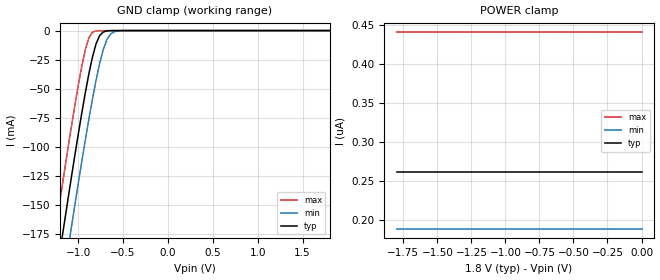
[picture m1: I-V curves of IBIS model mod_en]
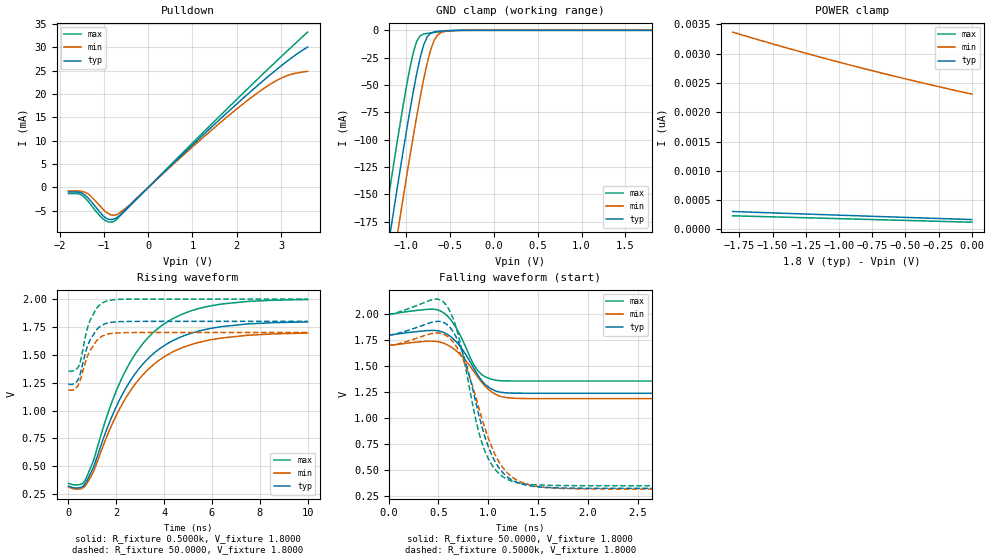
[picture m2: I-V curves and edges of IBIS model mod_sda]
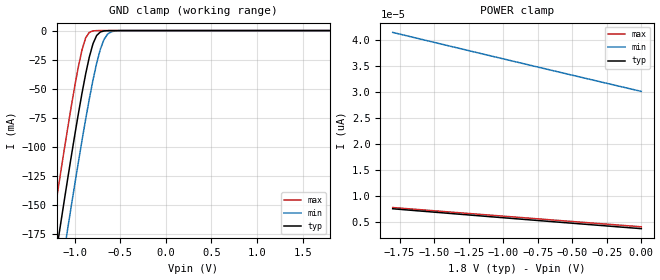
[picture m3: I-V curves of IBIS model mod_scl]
| IBIS (I/O, Buffer, Information, Specification) Model, officially
| electronic behavioral standard for Buffer structures of digital pins.
[IBIS ver]  4.0
[File name] m24c32_fd1_tssop8.ibs
[File Rev]  1.0
[Date]   2 March 2015
[Source]   CAD & Design Services (Catania) - STMicroelectronics
[Notes]
   (Note1)  This IBIS model includes the TSSOP8 package data
   (Note2)  This IBIS model has some Notes about the non-monotonicity
   of the I-V curves, but they are not indicative of problems
   inside the model;
[Copyright] (c) 2015 STMicroelectronics
|   Component M24C32
[Component] M24C32
[Manufacturer] STMicroelectronics
[Package]
| variable   typ   min   max
R_pkg   0.0   0.0   0.0
L_pkg   0.0H   0.0H   0.0H
C_pkg   0.0F   0.0F   0.0F
[Pin]   signal_name   model_name   R_pin   L_pin   C_pin
1   E1   mod_en   NA   NA   NA
2   E2   mod_en   NA   NA   NA
3   E3   mod_en   NA   NA   NA
4   VSS   GND   NA   NA   NA
5   SDA   mod_sda   NA   NA   NA
6   SCL   mod_scl   NA   NA   NA
7   WC   mod_wc   NA   NA   NA
8   VCC   POWER   NA   NA   NA
[Package Model]  182696_TSSOP8
[Define Package Model]  182696_TSSOP8
[Manufacturer]  STMicroelectronics
[OEM]  STMicroelectronics
[Description]  8 pin TSSOP package
[Number Of Pins]  8
[Pin Numbers]
|Pin Num   Terminal Name
1   | net1
2   | net2
3   | net3
4   | net4_GND
5   | net5
6   | net6
7   | net7
8   | net8_VDD
[Model Data]
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[End Model Data]
[End Package Model]
| Models and submodels in the file (4): mod_en (Input), mod_sda (I/O_open_drain), mod_scl (Input), mod_wc (Input)
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|   Model mod_en
[Model]   mod_en
Model_type Input
Vinl   =   0.540V
Vinh   =   1.260V
C_comp   1.763pF   1.683pF   1.933pF
[Temperature Range]  25.0000   85.0000   -40.0000
[Voltage Range]   1.8000V   1.7000V   2.0000V
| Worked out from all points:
|   GND clamp passes 1 mA (typ) near -0.71 V on its own axis
[GND_clamp]
|Voltage   I(typ)   I(min)   I(max)
-1.8V     -506.7mA   -549.3mA   -463.8mA
-1.28V    -230.6mA   -274mA     -186.5mA
-1.24V    -209.8mA   -253.3mA   -165.8mA
-1.16V    -168.9mA   -212.2mA   -124.8mA
-1.08V    -128.7mA   -171.8mA   -85.14mA
-920mV    -53.64mA   -94.29mA   -16.44mA
-840mV    -22.68mA   -58.76mA   -1.468mA
-800mV    -11.31mA   -42.6mA    -261.9uA
-720mV    -1.249mA   -16.25mA   -6.98uA
-680mV    -318.6uA   -7.797mA   -1.128uA
-600mV    -18.77uA   -1.043mA   -29.45nA
1.8V      3.674pA    30.76pA    3.627pA
[POWER_clamp]
|Voltage   I(typ)   I(min)   I(max)
-1.8V     261.2nA    189.1nA    440.6nA
-1.78V    261.2nA    189.1nA    440.6nA
-1.76V    261.2nA    189.1nA    440.6nA
0V        261.2nA    189.1nA    440.6nA
|   Model mod_sda
[Model]   mod_sda
Model_type I/O_open_drain
Polarity   Inverting
Vinl   =   0.540V
Vinh   =   1.260V
Vmeas  =   0.900V
Cref   =   10pF
Rref   =   1k
Vref   =   1.800V
C_comp   1.845pF   1.762pF   2.023pF
[Temperature Range]  25.0000   85.0000   -40.0000
[Voltage Range]   1.8000V   1.7000V   2.0000V
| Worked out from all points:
|   slope of the pulldown table from 0 to 0.27 V, typ, clamps not added: 109 ohm
|   GND clamp passes 1 mA (typ) near -0.65 V on its own axis
|   rising waveform, R_fixture 0.5000k, V_fixture 1.8000: 20-80 % time 2.25ns typ, 2.31ns min, 2.17ns max; typ from 0.322 V to 1.79 V
|   rising waveform, R_fixture 50.0000, V_fixture 1.8000: 20-80 % time 545ps typ, 565ps min, 512ps max; typ from 1.24 V to 1.8 V
|   falling waveform, R_fixture 50.0000, V_fixture 1.8000: 20-80 % time 225ps typ, 254ps min, 198ps max; typ from 1.8 V to 1.24 V
|   falling waveform, R_fixture 0.5000k, V_fixture 1.8000: 20-80 % time 266ps typ, 296ps min, 236ps max; typ from 1.8 V to 0.322 V
[Pulldown]
|Voltage   I(typ)   I(min)   I(max)
-1.8V     -956.6uA   -736.7uA   -1.299mA
-1.56V    -1.02mA    -766uA     -1.377mA
-1.38V    -2.037mA   -1.217mA   -2.706mA
-1.02V    -6.05mA    -4.667mA   -6.729mA
-900mV    -6.803mA   -5.579mA   -7.367mA
-780mV    -6.779mA   -5.962mA   -7.317mA
-660mV    -6.106mA   -5.539mA   -6.328mA
-480mV    -4.437mA   -4.234mA   -4.601mA
1.2V      10.89mA    10.37mA    11.4mA
2.4V      21.26mA    19.77mA    22.56mA
3.06V     26.48mA    23.66mA    28.53mA
3.6V      30.07mA    24.87mA    33.28mA
[GND_clamp]
|Voltage   I(typ)   I(min)   I(max)
-1.8V     -518.5mA   -561.2mA   -477.1mA
-1.28V    -237.2mA   -280.6mA   -194.5mA
-1.24V    -216mA     -259.5mA   -173.3mA
-1.16V    -174.3mA   -217.7mA   -131.6mA
-1.08V    -133.3mA   -176.5mA   -91.09mA
-920mV    -56.72mA   -97.5mA    -20.77mA
-840mV    -25.03mA   -61.28mA   -5.008mA
-800mV    -13.32mA   -44.79mA   -3.408mA
-720mV    -2.603mA   -17.83mA   -2.376mA
-680mV    -1.384mA   -9.107mA   -1.989mA
-600mV    -612.9uA   -1.891mA   -1.25mA
1.8V      166.6pA    2.361nA    109.5pA
[POWER_clamp]
|Voltage   I(typ)   I(min)   I(max)
-1.8V     304.6pA    3.37nA     231.1pA
-1.36V    269.7pA    3.079nA    204.3pA
-920mV    235.6pA    2.809nA    177.5pA
-480mV    202.2pA    2.561nA    150.8pA
0V        166.6pA    2.311nA    121.7pA
[Ramp]
| variable   typ   min   max
dV/dt_r   0.3370/0.5861n   0.3078/0.6032n   0.3862/0.5628n
dV/dt_f   0.3368/0.2838n   0.3075/0.2962n   0.3859/0.2619n
R_load = 50.0000
[Rising Waveform]
R_fixture= 0.5000k
V_fixture= 1.8000
V_fixture_min= 1.7000
V_fixture_max= 2.0000
|time   V(typ)   V(min)   V(max)
0s        321.8mV    314.6mV    346.1mV
700ps     344.7mV    324.2mV    376.4mV
1.05ns    494.1mV    454.1mV    554.7mV
1.75ns    912.3mV    841.1mV    1.038V
2.25ns    1.143V     1.059V     1.298V
2.95ns    1.376V     1.281V     1.555V
3.79ns    1.551V     1.451V     1.744V
4.79ns    1.668V     1.566V     1.867V
5.95ns    1.737V     1.635V     1.939V
10ns      1.795V     1.695V     1.996V
[Rising Waveform]
R_fixture= 50.0000
V_fixture= 1.8000
V_fixture_min= 1.7000
V_fixture_max= 2.0000
|time   V(typ)   V(min)   V(max)
0s        1.238V     1.187V     1.356V
220ps     1.24V      1.188V     1.359V
420ps     1.286V     1.234V     1.395V
520ps     1.352V     1.292V     1.461V
760ps     1.555V     1.467V     1.712V
920ps     1.638V     1.544V     1.815V
1.24ns    1.739V     1.64V      1.933V
1.62ns    1.784V     1.684V     1.983V
2.52ns    1.799V     1.699V     1.999V
10ns      1.8V       1.7V       2V
[Falling Waveform]
R_fixture= 50.0000
V_fixture= 1.8000
V_fixture_min= 1.7000
V_fixture_max= 2.0000
|time   V(typ)   V(min)   V(max)
0s        1.8V       1.7V       2V
420ps     1.844V     1.741V     2.049V
540ps     1.829V     1.725V     2.021V
620ps     1.786V     1.689V     1.95V
700ps     1.71V      1.629V     1.831V
840ps     1.505V     1.47V      1.542V
900ps     1.407V     1.387V     1.451V
1ns       1.3V       1.278V     1.385V
1.12ns    1.249V     1.21V      1.36V
10ns      1.238V     1.187V     1.356V
[Falling Waveform]
R_fixture= 0.5000k
V_fixture= 1.8000
V_fixture_min= 1.7000
V_fixture_max= 2.0000
|time   V(typ)   V(min)   V(max)
0s        1.8V       1.7V       2V
460ps     1.928V     1.818V     2.145V
580ps     1.905V     1.794V     2.086V
740ps     1.635V     1.579V     1.638V
880ps     1.132V     1.183V     962.3mV
980ps     780.3mV    862.7mV    650.1mV
1.14ns    479.7mV    530.2mV    439.1mV
1.32ns    369.1mV    386.4mV    371.9mV
1.98ns    324mV      317.4mV    347.9mV
10ns      321.8mV    314.6mV    346.1mV
|   Model mod_scl
[Model]   mod_scl
Model_type Input
Vinl   =   0.540V
Vinh   =   1.260V
C_comp   1.763pF   1.683pF   1.933pF
[Temperature Range]  25.0000   85.0000   -40.0000
[Voltage Range]   1.8000V   1.7000V   2.0000V
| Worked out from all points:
|   GND clamp passes 1 mA (typ) near -0.71 V on its own axis
[GND_clamp]
|Voltage   I(typ)   I(min)   I(max)
-1.8V     -506.7mA   -549.3mA   -463.8mA
-1.28V    -230.6mA   -274mA     -186.5mA
-1.24V    -209.8mA   -253.3mA   -165.8mA
-1.16V    -168.9mA   -212.2mA   -124.8mA
-1.08V    -128.7mA   -171.8mA   -85.14mA
-920mV    -53.64mA   -94.29mA   -16.44mA
-840mV    -22.68mA   -58.76mA   -1.468mA
-800mV    -11.31mA   -42.6mA    -261.9uA
-720mV    -1.249mA   -16.25mA   -6.98uA
-680mV    -318.6uA   -7.797mA   -1.128uA
-600mV    -18.77uA   -1.043mA   -29.45nA
1.8V      3.674pA    30.76pA    3.627pA
[POWER_clamp]
|Voltage   I(typ)   I(min)   I(max)
-1.8V     7.509pA    41.51pA    7.748pA
-940mV    5.652pA    36.04pA    5.962pA
-440mV    4.594pA    32.89pA    4.934pA
0V        3.674pA    30.14pA    4.034pA
